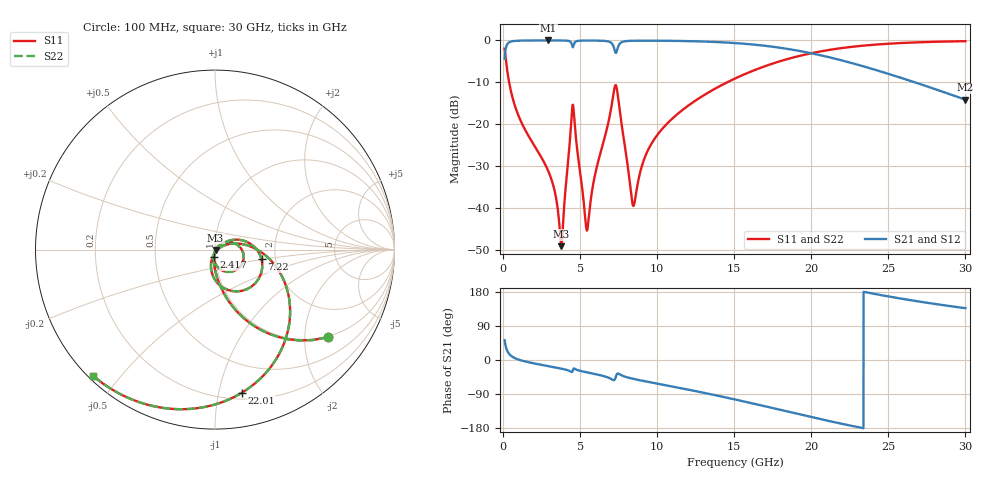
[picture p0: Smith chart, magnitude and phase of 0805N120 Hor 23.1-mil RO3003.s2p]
# GHz S MA R 50
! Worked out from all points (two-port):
!   3201 points, 100 MHz to 30 GHz, reference 50 ohm
!   highest |S21| = -0.02 dB at 2.941 GHz (marker M1); lowest = -14.1 dB at 30 GHz (marker M2)
!   |S21| within 3 dB of the highest: 131.4 MHz to 19.93 GHz (19.8 GHz wide, 197 % of centre)
!   lowest |S11| = -49.1 dB at 3.781 GHz (marker M3), VSWR 1.01, Z = 50.3 - j0.164 ohm
!   |S11| at or under -10 dB: 392.7 MHz to 14.54 GHz (14.15 GHz wide, 189 % of centre)
!   |S22| runs from -49.1 to -0.2 dB; largest |S21 - S12| = 0
!   S11 on the Smith chart (normalised r, x): 100 MHz: 0.97, -2.59; 2.417 GHz: 0.98, -0.08; 7.22 GHz: 1.69, -0.19; 22.01 GHz: 0.25, -1.18; 30 GHz: 0.01, -0.43
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0.1  0.7957 -37.8  0.6051 52.1  0.6051 52.1  0.7957 -37.8
0.32425  0.3748 -69.9  0.9265 20.0  0.9265 20.0  0.3748 -69.9
0.5578437  0.2275 -80.1  0.973 9.8  0.973 9.8  0.2275 -80.1
2.41725  0.04231 -99.9  0.9973 -12.2  0.9973 -12.2  0.04231 -99.9
2.9405  0.02739 -102.0  0.9975 -16.3  0.9975 -16.3  0.02739 -102.0
3.781438  0.003514 -27.6  0.9964 -22.8  0.9964 -22.8  0.003514 -27.6
4.500906  0.164 -12.3  0.8423 -30.0  0.8423 -30.0  0.164 -12.3
4.622375  0.116 -74.2  0.9236 -22.6  0.9236 -22.6  0.116 -74.2
5.089563  0.02003 -98.2  0.9924 -29.5  0.9924 -29.5  0.02003 -98.2
5.351187  0.006911 -67.8  0.9942 -31.8  0.9942 -31.8  0.006911 -67.8
5.491344  0.005858 -8.1  0.9945 -33.0  0.9945 -33.0  0.005858 -8.1
5.939844  0.02365 39.2  0.9938 -36.8  0.9938 -36.8  0.02365 39.2
7.219938  0.2646 -11.6  0.7854 -52.8  0.7854 -52.8  0.2646 -11.6
7.434844  0.2289 -74.4  0.8105 -35.8  0.8105 -35.8  0.2289 -74.4
8.443969  0.01062 -45.7  0.9891 -49.7  0.9891 -49.7  0.01062 -45.7
9.163438  0.03869 23.5  0.9917 -55.7  0.9917 -55.7  0.03869 23.5
10.06978  0.07707 22.5  0.9905 -62.9  0.9905 -62.9  0.07707 22.5
15.05  0.3508 -15.3  0.9286 -104.1  0.9286 -104.1  0.3508 -15.3
20.03956  0.7048 -61.7  0.6994 -150.9  0.6994 -150.9  0.7048 -61.7
22.01109  0.8108 -79.3  0.5748 -168.6  0.5748 -168.6  0.8108 -79.3
25.01978  0.9124 -103.0  0.3981 167.6  0.3981 167.6  0.9124 -103.0
30  0.9777 -133.8  0.1963 136.7  0.1963 136.7  0.9777 -133.8
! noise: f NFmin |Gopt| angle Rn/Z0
0.1  0.00068  0.9095  0.9497  0.001652
3.417  0.007024  0.7306  20.71  0.005032
6.743  0.02609  0.8513  40.03  0.03304
10.06  0.01836  0.7185  58.15  0.00994
13.39  0.02184  0.7019  74.57  0.009248
16.7  0.02771  0.7175  89.58  0.01003
20.03  0.03568  0.7455  103.5  0.01117
23.35  0.04677  0.7815  116.6  0.01261
26.67  0.06319  0.8229  129.2  0.01433
30  0.08909  0.8661  141.7  0.01605
